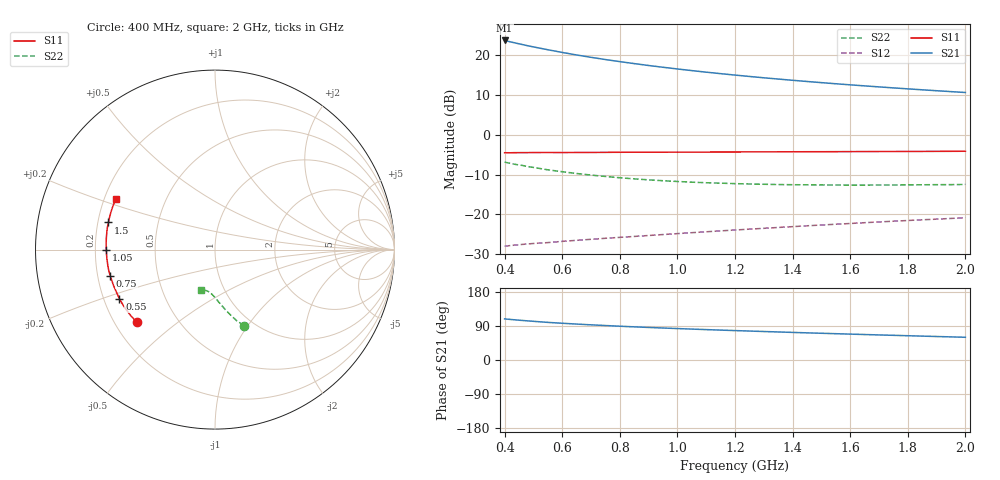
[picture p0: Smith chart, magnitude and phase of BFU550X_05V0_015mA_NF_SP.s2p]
! Filename:  P:\Prog\Test\Noise\ATS_data\Testdata_Net\BFU550X attenuator noise\BFU550X_APG2013_44_C05_05p0V_015mA_NF_CM01_D.sf
! Date/Time: Fri 26/Jul/2013 14:34:20
! BFU550X_APG2013_44_C05_05p0V_1to35mA_NF_CM01_Bias6_R.sf
! Noise Parameter Data File
! BFU550X_APG2013_44_C05_05p0V_1to35mA_NF_CM01
! Date/time: Mon Jul 22 09:12:23 2013
! VAR V_out= 5.001000
! VAR I_out= 15.000000
! VAR V_in= 0.825500
! VAR I_in= 0.166600
! Device data file deembeded for feedlines and parallel
! Original file: \BFU550X attenuator noise\BFU550X_APG2013_44_C05_05p0V_015mA_NF_CM01_R.sf
! Feed-files: PR005V01_100713_Feed1.s2p, PR005V01_100713_Feed2.s2p
! Parallel-file: PR005V01_100713_Par.s2p
# MHz S MA R 50
!  Freq-MHz  S11-mag  S11-arg  S21-mag  S21-arg  S12-mag  S12-arg  S22-mag  S22-arg
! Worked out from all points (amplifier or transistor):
!   37 points, 400 MHz to 2 GHz, reference 50 ohm
!   highest |S21| = 23.7 dB at 400 MHz (marker M1)
!   |S21| within 3 dB of that: start of sweep to 599.6 MHz
!   unconditionally stable (mu >= 1): 1.665 GHz to end of sweep
!   at 500 MHz: K = 0.54, MSG = 24.7 dB, |S12| = -27.3 dB
!   at 1.1 GHz: K = 0.88, MSG = 20.0 dB, |S12| = -24.4 dB
!   at 2 GHz: K = 1.04, MAG = 14.6 dB, |S12| = -20.8 dB
!   lowest NFmin = 0.91 dB at 480 MHz
!   S11 on the Smith chart (normalised r, x): 400 MHz: 0.29, -0.36; 550 MHz: 0.26, -0.23; 750 MHz: 0.25, -0.11; 1.05 GHz: 0.25, -0.00; 1.5 GHz: 0.24, +0.12; 2 GHz: 0.25, +0.23
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400  0.5952 -137.1  15.28 108.4  0.03995 44.3  0.4534 -69.3
420  0.5944 -139.5  14.67 107.0  0.04065 44.1  0.4375 -70.8
440  0.5962 -141.8  14.13 105.7  0.04133 43.9  0.4235 -71.8
460  0.5966 -144.0  13.61 104.4  0.04199 43.8  0.4129 -73.2
500  0.5983 -148.1  12.68 102.1  0.04315 43.5  0.3893 -75.2
550  0.5991 -152.8  11.69 99.3  0.0443 43.6  0.363 -77.7
600  0.5981 -156.5  10.81 97.0  0.04589 43.9  0.3439 -79.8
650  0.5996 -160.1  10.04 94.8  0.0473 44.2  0.3264 -81.6
700  0.6003 -163.1  9.385 92.8  0.04872 44.6  0.312 -83.3
750  0.6016 -166.1  8.8 90.9  0.05017 45.0  0.2996 -85.0
800  0.6031 -168.7  8.289 89.2  0.05153 45.4  0.2888 -86.6
850  0.6038 -171.3  7.827 87.5  0.05292 45.9  0.2795 -87.9
900  0.6036 -173.6  7.41 85.9  0.05437 46.5  0.2717 -89.2
950  0.6045 -175.7  7.042 84.4  0.05589 47.0  0.2648 -90.4
1050  0.6055 -179.7  6.393 81.6  0.05899 47.9  0.2541 -92.7
1100  0.6066 178.4  6.111 80.2  0.06055 48.3  0.2499 -93.7
1200  0.6082 174.9  5.617 77.6  0.06373 49.0  0.2436 -95.8
1350  0.611 170.1  5.006 74.0  0.0686 50.0  0.2372 -98.5
1500  0.6131 165.7  4.515 70.5  0.07363 50.7  0.2346 -101.1
1600  0.6145 162.9  4.236 68.3  0.07695 51.1  0.2336 -102.5
1750  0.6167 159.0  3.878 65.1  0.08219 51.5  0.2344 -105.0
2000  0.6213 153.1  3.394 60.0  0.0908 51.8  0.2378 -108.5
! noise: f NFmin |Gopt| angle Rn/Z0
400  0.9735  0.2066  177.8  0.073
460  0.9108  0.2202  -178.2  0.0705
600  0.9335  0.2468  -178.5  0.0648
800  0.9612  0.2665  -176.8  0.0627
1000  0.9897  0.2902  -174.3  0.0596
1200  1.011  0.3168  -173.3  0.0575
1400  1.033  0.3299  -170.2  0.0601
1600  1.094  0.3421  -161.7  0.0668
1800  1.063  0.3749  -167.7  0.0555
2000  1.14  0.3896  -163.9  0.0589
